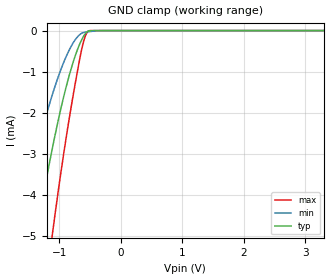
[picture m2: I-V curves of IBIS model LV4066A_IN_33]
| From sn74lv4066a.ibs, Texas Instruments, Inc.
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[Model]   LV4066A_IN_33
Model_type  Input
Vinl = 0.9
Vinh = 2.52
| variable   typ   min   max
C_comp   1.27pF   0.81pF   1.46pF
[Temperature Range]   40   100   -40
| Ambient temperature   25   85   -40
[Voltage range]   3.3   3   3.6
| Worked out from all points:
|   GND clamp passes 1 mA (typ) near -0.82 V on its own axis
[GND Clamp]
| LV4066A_IN_33
|   Voltage   I(typ)   I(min)   I(max)
-3.3V     -27.15mA   -18.54mA   -40.03mA
-1.675V   -7.856mA   -4.918mA   -12.36mA
-1.365V   -4.931mA   -2.922mA   -8.068mA
-1.225V   -3.748mA   -2.134mA   -6.301mA
-1.105V   -2.818mA   -1.528mA   -4.89mA
-965mV    -1.849mA   -918.5uA   -3.379mA
-850mV    -1.162mA   -512.6uA   -2.26mA
-725mV    -552.3uA   -193.2uA   -1.168mA
-625mV    -195.3uA   -58.14uA   -394.4uA
-570mV    -65.36uA   -37.36uA   -114.8uA
-510mV    -6.292uA   -25.2uA    -1.454uA
3.3V      13.4pA     149.4pA    9.907pA
